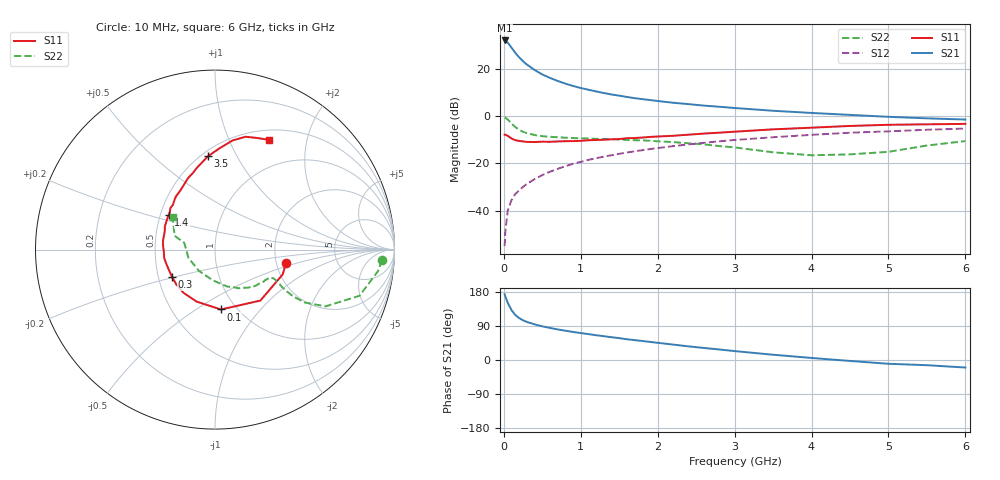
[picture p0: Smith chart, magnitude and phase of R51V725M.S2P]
! SIEMENS Small Signal Semiconductors
! BFR183
! Si NPN RF Bipolar Junction Transistor in SOT23
! VCE = 1.75 V  IC = 25 mA
! Common Emitter S-Parameters:  May  1996
# GHz  S  MA  R  50
!  f  S11  S21  S12  S22
! GHz  MAG  ANG  MAG  ANG  MAG  ANG  MAG  ANG
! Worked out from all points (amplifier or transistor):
!   36 points, 10 MHz to 6 GHz, reference 50 ohm
!   highest |S21| = 31.8 dB at 10 MHz (marker M1)
!   |S21| within 3 dB of that: start of sweep to 98.43 MHz
!   unconditionally stable (mu >= 1): 399.6 MHz to 2.436 GHz
!   at 250 MHz: K = 0.89, MSG = 26.5 dB, |S12| = -29.9 dB
!   at 1.4 GHz: K = 1.06, MAG = 11.3 dB, |S12| = -16.6 dB
!   at 6 GHz: K = 0.92, MSG = 1.9 dB, |S12| = -5.3 dB
!   S11 on the Smith chart (normalised r, x): 10 MHz: 2.26, -0.40; 100 MHz: 0.85, -0.64; 300 MHz: 0.59, -0.20; 1.4 GHz: 0.55, +0.24; 3.5 GHz: 0.54, +0.77; 6 GHz: 0.62, +1.42
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0.01  0.4031 -10.5  39.02 173.7  0.0018 85.1  0.9322 -3.6
0.02  0.4017 -20.1  38.54 167.5  0.0037 83.7  0.9164 -7.5
0.05  0.3802 -48.3  35.17 151.2  0.01 74.6  0.8455 -17.7
0.1  0.3353 -84.3  27.41 131.5  0.017 69.2  0.6922 -27.2
0.15  0.3074 -109.5  21.33 118.5  0.0228 68.2  0.5813 -30.5
0.2  0.2979 -126.4  17.17 110.5  0.027 68.8  0.5095 -30.9
0.25  0.29 -137.9  14.19 104.7  0.0321 69.4  0.4624 -30.2
0.3  0.2841 -147.0  12.1 100.4  0.037 70.5  0.434 -29.4
0.4  0.2818 -161.6  9.307 94.1  0.0466 71.5  0.3963 -27.6
0.5  0.2871 -170.4  7.498 88.8  0.0567 72.3  0.3746 -26.5
0.6  0.2851 -177.5  6.337 84.6  0.0668 72.5  0.3632 -26.2
0.7  0.2903 175.8  5.472 80.7  0.0769 72.2  0.3559 -26.4
0.8  0.294 170.2  4.802 77.3  0.0872 71.4  0.3477 -26.7
0.9  0.2951 164.5  4.284 74.0  0.0982 71.1  0.342 -27.2
1.1  0.3074 155.5  3.565 68.3  0.1186 69.7  0.3342 -29.7
1.4  0.3222 143.3  2.835 60.1  0.1486 66.9  0.3236 -33.6
1.7  0.3422 133.3  2.371 52.5  0.1797 63.7  0.3084 -38.4
2.2  0.3818 120.4  1.898 40.7  0.2311 57.8  0.2817 -48.8
3.5  0.5222 94.2  1.286 13.9  0.3558 40.5  0.1714 -94.2
4.5  0.6156 80.9  1.053 -2.5  0.4435 27.2  0.155 -162.4
5.5  0.6663 68.8  0.891 -13.7  0.5119 15.1  0.238 161.1
6  0.681 63.8  0.84 -19.9  0.543 7.3  0.2953 142.7
